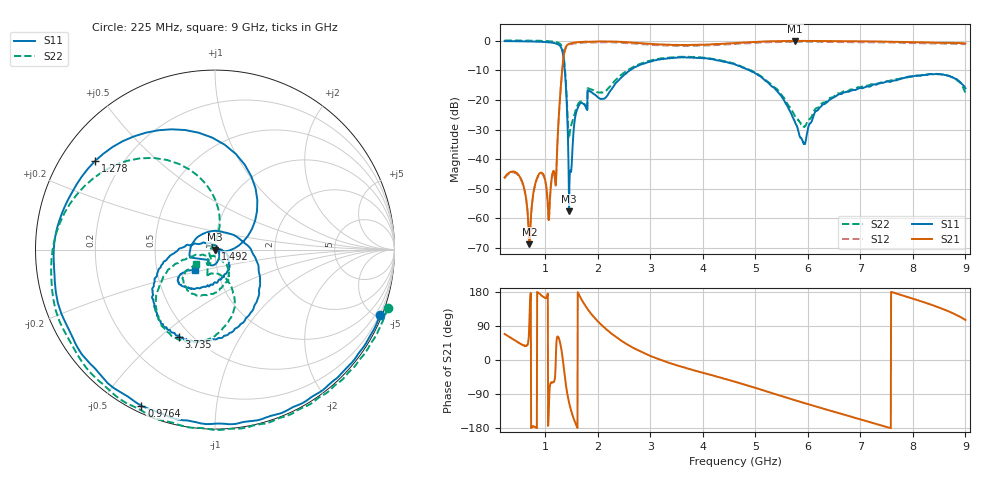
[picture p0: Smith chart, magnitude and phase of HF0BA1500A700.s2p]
!Agilent Technologies,E8358A,US41080443,A.07.50.56
!Agilent E8358A: A.07.50.56
!Date: Wednesday, June 22, 2016 13:08:38
!Correction: S11(Full 2 Port(1,2))
!S21(Full 2 Port(1,2))
!S12(Full 2 Port(1,2))
!S22(Full 2 Port(1,2))
!S2P File: Measurements: S11, S21, S12, S22:
# Hz S  dB  R 50
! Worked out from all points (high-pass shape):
!   1601 points, 225 MHz to 9 GHz, reference 50 ohm
!   highest |S21| = 0.01 dB at 5.759 GHz (marker M1); lowest = -68.7 dB at 696.7 MHz (marker M2)
!   |S21| within 3 dB of the highest: 1.374 GHz to end of sweep
!   lowest |S11| = -57.6 dB at 1.454 GHz (marker M3), VSWR 1.00, Z = 49.9 + j0.00567 ohm
!   |S11| at or under -10 dB: 1.371 GHz to 2.607 GHz (1.235 GHz wide, 62.1 % of centre); 4.894 GHz to end of sweep
!   |S22| runs from -33.1 to 0.1 dB; largest |S21 - S12| = 0.038
!   S11 on the Smith chart (normalised r, x): 225 MHz: 0.13, -5.24; 976.4 MHz: 0.03, -0.63; 1.278 GHz: 0.10, +0.33; 1.492 GHz: 1.01, +0.01; 3.735 GHz: 0.43, -0.58; 9 GHz: 0.78, -0.18
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2.25e8  -0.08 -21.6  -46.19 68.6  -46.50 69.4  0.15 -18.8
5.211562e8  -0.12 -51.8  -46.07 43.4  -46.42 43.3  0.11 -44.7
6.966562e8  -0.20 -72.4  -68.73 99.5  -69.39 99.1  0.05 -62.5
8.282812e8  -0.26 -90.2  -47.07 -179.1  -47.45 -178.1  0.03 -78.0
9.763594e8  -0.34 -115.2  -45.69 165.5  -45.97 165.5  0.01 -99.1
1.086047e9  -0.52 -138.8  -54.24 -69.7  -54.43 -70.4  -0.12 -118.9
1.201219e9  -0.91 -175.1  -48.45 8.8  -48.76 9.1  -0.40 -149.1
1.278e9  -1.61 143.5  -19.64 47.8  -19.96 48.1  -0.94 177.1
1.36575e9  -8.79 49.5  -3.57 -36.8  -3.90 -36.7  -7.62 102.4
1.4535e9  -57.63 177.5  -1.00 -112.8  -1.32 -112.6  -32.65 166.3
1.491891e9  -44.31 59.2  -0.78 -133.6  -1.10 -133.4  -28.50 -149.1
1.579641e9  -24.81 -70.1  -0.51 -168.9  -0.84 -168.6  -23.33 -108.6
1.689328e9  -20.87 -104.4  -0.36 159.7  -0.68 160.0  -20.49 -115.1
2.139047e9  -19.35 66.3  -0.18 83.7  -0.49 83.9  -17.15 -80.6
3.153656e9  -6.33 -83.1  -1.14 2.4  -1.47 2.5  -6.05 -93.7
3.735e9  -5.58 -112.5  -1.36 -23.5  -1.69 -23.4  -5.39 -114.5
4.6125e9  -7.99 -149.0  -0.75 -57.4  -1.07 -57.3  -7.80 -142.8
5.758734e9  -27.65 120.5  0.01 -106.4  -0.32 -106.4  -25.53 -142.4
5.923266e9  -34.81 48.2  -0.02 -113.1  -0.33 -113.1  -29.05 -105.8
6.076828e9  -27.02 -10.8  -0.02 -119.4  -0.34 -119.5  -25.40 -64.9
7.541156e9  -13.77 -101.0  -0.27 -178.5  -0.59 -178.6  -13.51 -79.4
9e9  -16.02 -134.9  -0.85 105.7  -1.15 105.5  -17.44 -143.5
